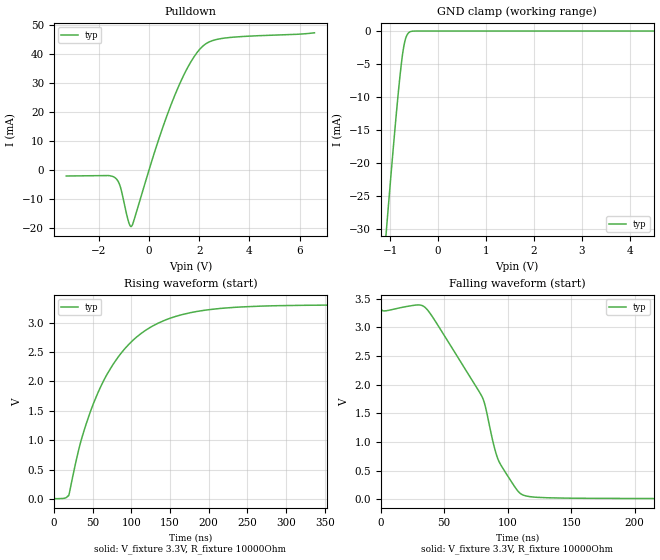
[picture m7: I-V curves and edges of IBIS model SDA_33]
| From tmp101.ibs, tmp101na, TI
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|   SDA 3.3 V Model
[Model]   SDA_33
Model_type   I/O_open_drain
Polarity   Non-Inverting
Enable   Active-Low
Vinl = 0.66
Vinh = 2.31
Vmeas = 1.65
Vref = 1.65
Cref = 15pF
Rref = 10000
|   typ   min   max
C_comp   4.96pf   NA   NA
[Voltage Range]   3.3   NA   NA
[Temperature Range]   27   NA   NA
[Pullup Reference]   3.3   NA   NA
[Pulldown Reference]   0   NA   NA
[Power Clamp Reference]   3.3   NA   NA
[GND Clamp Reference]   0   NA   NA
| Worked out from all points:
|   slope of the pulldown table from 0 to 0.495 V, typ, clamps not added: 37.1 ohm
|   GND clamp passes 1 mA (typ) near -0.67 V on its own axis
|   falling waveform, V_fixture 3.3V, R_fixture 10000Ohm: 20-80 % time 36.9ns typ, NA min, NA max; typ from 3.3 V to 0.012 V
|   rising waveform, V_fixture 3.3V, R_fixture 10000Ohm: 20-80 % time 68.6ns typ, NA min, NA max; typ from 0.012 V to 3.3 V
[Pulldown]
|   Voltage   I(typ)   I(min)   I(max)
-3.3V     -2.116mA   NA         NA
-1.348V   -2.755mA   NA         NA
-1.155V   -5.541mA   NA         NA
-830.4mV  -17.5mA    NA         NA
-706.6mV  -19.52mA   NA         NA
326.9mV   8.997mA    NA         NA
897.1mV   22.92mA    NA         NA
1.508V    34.8mA     NA         NA
2.055V    41.91mA    NA         NA
2.42V     44.19mA    NA         NA
2.981V    45.39mA    NA         NA
6.59V     47.23mA    NA         NA
[GND Clamp]
|   Voltage   I(typ)   I(min)   I(max)
-3.3V     -232.4mA   NA         NA
-1.085V   -30.46mA   NA         NA
-1.075V   -29.57mA   NA         NA
-961.6mV  -19.74mA   NA         NA
-861.6mV  -11.55mA   NA         NA
-804mV    -7.266mA   NA         NA
-762.3mV  -4.566mA   NA         NA
-721.5mV  -2.49mA    NA         NA
-683.8mV  -1.234mA   NA         NA
-633.8mV  -410.9uA   NA         NA
-584.7mV  -107.4uA   NA         NA
6.59V     0A         NA         NA
[POWER Clamp]
|   SCR cell for ESD function. Effects occurr above VDD x 2
|   Voltage   I(typ)   I(min)   I(max)
-3.3V     0A         0A         0A
0V        0A         0A         0A
6.6V      0A         0A         0A
[Ramp]
R_load = 10000
|   typ   min   max
dV/dt_r   1.97308/6.86366e-008 NA   NA
dV/dt_f   1.97308/3.68572e-008 NA   NA
[Falling Waveform]
V_fixture = 3.3V
R_fixture = 10000Ohm
C_fixture = 0F
|   Time   V(typ)   V(min)   V(max)
0s        3.3V       NA         NA
29.82ns   3.388V     NA         NA
37.71ns   3.277V     NA         NA
80.12ns   1.773V     NA         NA
82.73ns   1.588V     NA         NA
89.77ns   881mV      NA         NA
93.84ns   628.3mV    NA         NA
108.4ns   133.6mV    NA         NA
117.9ns   45.97mV    NA         NA
1.197us   11.54mV    NA         NA
[Rising Waveform]
V_fixture = 3.3V
R_fixture = 10000Ohm
C_fixture = 0F
|   Time   V(typ)   V(min)   V(max)
0s        11.54mV    NA         NA
19.13ns   59.63mV    NA         NA
33.2ns    895.6mV    NA         NA
45.91ns   1.437V     NA         NA
63.55ns   1.993V     NA         NA
83.21ns   2.417V     NA         NA
123.2ns   2.908V     NA         NA
176.3ns   3.168V     NA         NA
320.6ns   3.293V     NA         NA
1.197us   3.3V       NA         NA
